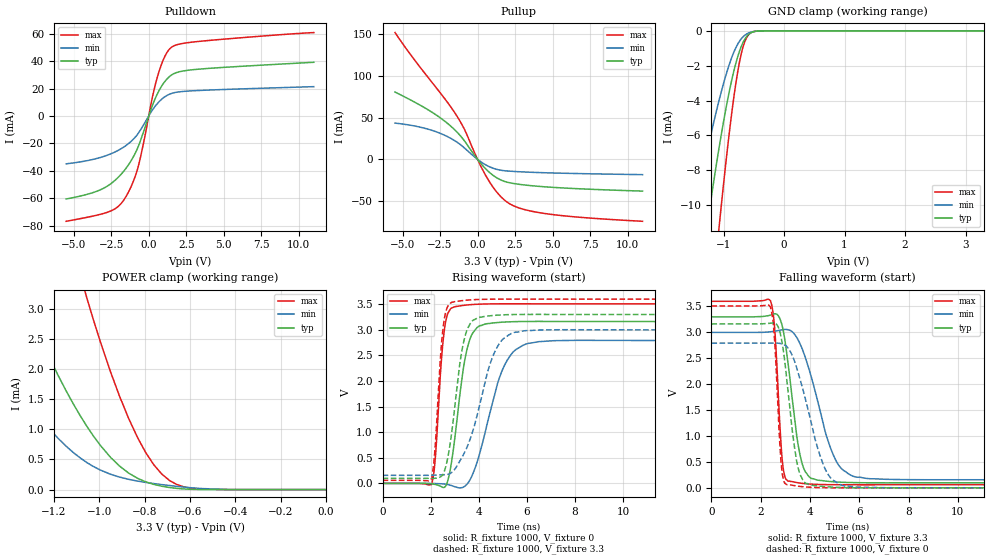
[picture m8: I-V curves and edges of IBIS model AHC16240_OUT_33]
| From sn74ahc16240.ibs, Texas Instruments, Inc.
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[Model]   AHC16240_OUT_33
Model_type  3-state
Enable   Active-Low
Vref =   0
Rref =   1000
Cref =   50p
Vmeas =   1.65
| variable   typ   min   max
C_comp   2.89pF   2.36pF   3.15pF
| C_pullup   3.89pF   2.55pF   4.82pF
| C_pulldown   3.68pF   2.92pF   4.78pF
| C_tri-state   2.89pF   2.36pF   3.15pF
[Temperature Range]   40   100   -40
| Ambient temperature   25   85   -40
[Voltage range]   3.3   3   3.6
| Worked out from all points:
|   slope of the pulldown table from 0 to 0.495 V, typ, clamps not added: 34.7 ohm
|   slope of the pullup table from 0 to 0.495 V, typ, clamps not added: 47.1 ohm
|   GND clamp passes 1 mA (typ) near -0.72 V on its own axis
|   POWER clamp passes 1 mA (typ) near -1.05 V on its own axis
|   rising waveform, R_fixture 1000, V_fixture 0: 20-80 % time 534ps typ, 978ps min, 297ps max; typ from 0 V to 3.16 V
|   falling waveform, R_fixture 1000, V_fixture 3.3: 20-80 % time 516ps typ, 1ns min, 241ps max; typ from 3.3 V to 0.097 V
|   rising waveform, R_fixture 1000, V_fixture 3.3: 20-80 % time 528ps typ, 1.02ns min, 289ps max; typ from 0.097 V to 3.3 V
|   falling waveform, R_fixture 1000, V_fixture 0: 20-80 % time 467ps typ, 945ps min, 225ps max; typ from 3.16 V to 0 V
[GND Clamp]
| AHC16240_OUT_33
|   Voltage   I(typ)   I(min)   I(max)
-5.5V     -169.3mA   -111.2mA   -212.8mA
-1.515V   -17.63mA   -11.11mA   -28.08mA
-1.265V   -11.08mA   -6.838mA   -18.23mA
-1.07V    -6.632mA   -3.938mA   -11.15mA
-895mV    -3.319mA   -1.829mA   -5.576mA
-830mV    -2.316mA   -1.23mA    -3.824mA
-775mV    -1.597mA   -824.7uA   -2.548mA
-715mV    -968.7uA   -494.7uA   -1.44mA
-665mV    -580uA     -303.9uA   -786.7uA
-610mV    -290.9uA   -166.7uA   -345.5uA
-550mV    -116.5uA   -78.88uA   -117.1uA
3.3V      12.3nA     24.67nA    59.73nA
[POWER Clamp]
| AHC16240_OUT_33
|   Voltage   I(typ)   I(min)   I(max)
-5.5V     86.69mA    55.4mA     139.9mA
-1.62V    6.126mA    3.297mA    12.9mA
-1.585V   5.725mA    3.057mA    12.18mA
-1.34V    3.216mA    1.58mA     7.527mA
-1.18V    1.886mA    846.3uA    4.928mA
-1.055V   1.053mA    450.5uA    3.186mA
-950mV    534.8uA    254.5uA    1.952mA
-870mV    273.4uA    170.2uA    1.178mA
-795mV    128.8uA    119.3uA    613.8uA
-690mV    34.71uA    67.53uA    150.6uA
-555mV    1.833uA    18.6uA     9.101uA
-95.1fV   12.3nA     1.801nA    93.24nA
[Pulldown]
| AHC16240_OUT_33
|   Voltage   I(typ)   I(min)   I(max)
-5.5V     -60.51mA   -34.9mA    -76.79mA
-3.03V    -52.82mA   -29.61mA   -71.14mA
-2.135V   -45.78mA   -25.64mA   -66.83mA
-1.53V    -38.35mA   -21.63mA   -59.01mA
-1.055V   -30.36mA   -17.26mA   -48.46mA
-695mV    -22.17mA   -12.58mA   -36.63mA
250mV     7.835mA    4.39mA     13.96mA
645mV     17.64mA    9.881mA    30.94mA
1.085V    25.28mA    14.08mA    43.67mA
1.505V    29.74mA    16.39mA    50mA
3.21V     34.02mA    18.52mA    54.22mA
11V       39.14mA    21.38mA    60.82mA
[Pullup]
| AHC16240_OUT_33
|   Voltage   I(typ)   I(min)   I(max)
-5.5V     80.62mA    43.42mA    151.9mA
-3.57V    62.27mA    37.46mA    104.4mA
-2.06V    43.96mA    27.73mA    69.66mA
-1.44V    33.92mA    21.41mA    53.71mA
-965mV    24.34mA    15.06mA    39.2mA
65mV      -1.523mA   -905.6uA   -2.508mA
670mV     -13.63mA   -7.794mA   -23.21mA
1.29V     -22.22mA   -12.06mA   -39.41mA
1.905V    -27.04mA   -13.84mA   -50.37mA
2.865V    -30.15mA   -14.95mA   -58.8mA
4.475V    -32.91mA   -16.07mA   -64.91mA
11V       -38.08mA   -18.35mA   -74.25mA
[Ramp]
| AHC16240_OUT_33
| variable   typ   min   max
dV/dt_r   1.95/5.66E-10   1.73/1.05E-09   2.12/3.01E-10
dV/dt_f   1.96/5.49E-10   1.74/1.05E-09   2.15/2.51E-10
R_load = 1000
[Rising Waveform]
| AHC16240_OUT_33
R_fixture =   1000
C_fixture =   0
L_fixture =   0
V_fixture =   0
V_fixture_min = 0
V_fixture_max = 0
|   Time   V(typ)   V(min)   V(max)
0s        183.9pV    418.7pV    74.68pV
2.035ns   -9.999mV   -1.273mV   -21.82mV
2.185ns   -20.76mV   -3.235mV   456.9mV
2.595ns   -67.12mV   -14.03mV   3.084V
3.225ns   1.774V     -87.3mV    3.47V
3.535ns   2.665V     -1.691mV   3.488V
3.94ns    3.049V     429.5mV    3.501V
5.095ns   3.154V     2.331V     3.51V
6.465ns   3.166V     2.768V     3.51V
50ns      3.163V     2.791V     3.509V
[Falling Waveform]
| AHC16240_OUT_33
R_fixture =   1000
C_fixture =   0
L_fixture =   0
V_fixture =   3.3
V_fixture_min = 3
V_fixture_max = 3.6
|   Time   V(typ)   V(min)   V(max)
0s        3.3V       3V         3.6V
2.395ns   3.334V     3.012V     3.613V
2.565ns   3.358V     3.022V     3.09V
2.815ns   3.219V     3.045V     917.2mV
2.925ns   3.009V     3.053V     337.2mV
3.605ns   614.3mV    2.77V      90.19mV
4.01ns    195mV      2.21V      71.78mV
5.03ns    113.4mV    546mV      59.76mV
6.305ns   96.85mV    180.2mV    58.2mV
50ns      97.11mV    157mV      59.03mV
[Rising Waveform]
| AHC16240_OUT_33
R_fixture =   1000
C_fixture =   0
L_fixture =   0
V_fixture =   3.3
V_fixture_min = 3
V_fixture_max = 3.6
|   Time   V(typ)   V(min)   V(max)
0s        97.11mV    157mV      59.03mV
2.035ns   98.67mV    159mV      93.1mV
2.17ns    99.57mV    161.1mV    618.7mV
2.54ns    203.5mV    169.2mV    3.126V
3.045ns   1.679V     304.6mV    3.556V
3.345ns   2.708V     545.6mV    3.573V
3.7ns     3.159V     947.3mV    3.588V
4.705ns   3.286V     2.608V     3.6V
5.885ns   3.302V     2.982V     3.601V
50ns      3.3V       3V         3.6V
[Falling Waveform]
| AHC16240_OUT_33
R_fixture =   1000
C_fixture =   0
L_fixture =   0
V_fixture =   0
V_fixture_min = 0
V_fixture_max = 0
|   Time   V(typ)   V(min)   V(max)
0s        3.163V     2.791V     3.509V
2.395ns   3.177V     2.793V     3.487V
2.555ns   3.18V      2.794V     2.91V
2.835ns   2.887V     2.781V     442.1mV
3.07ns    2.033V     2.72V      59.05mV
3.44ns    568.2mV    2.347V     36.69mV
3.705ns   152.8mV    1.911V     20.44mV
4.61ns    22.41mV    367.3mV    2.34mV
5.425ns   3.894mV    32.61mV    -248.8uV
50ns      60.41nV    35.46nV    3.68nV
